(* Logix 5000 AddOnInstructionDefinition export AMP_Point_to_Point_FC; software revision 20.04 *)

TYPE AMP_Status_Word :   // Applied Motion Input Assembly Status Word
STRUCT
   Enabled : BOOL;   // Motor Enabled (Motor Disabled if this bit = 0)
   Sampling : BOOL;   // Sampling (for Quick Tuner)
   Drive_Fault : BOOL;   // Drive Fault (check Alarm Code)
   In_Position : BOOL;   // In Position (motor is in position)
   Moving : BOOL;   // Moving (motor is moving)
   Jogging : BOOL;   // Jogging (currently in jog mode)
   Stopping : BOOL;   // Stopping (in the process of stopping from a stop command)
   Waiting : BOOL;   // Waiting (for an input; executing a WI command)
   Saving : BOOL;   // Saving (parameter data is being saved)
   Alarm_Present : BOOL;   // Alarm present (check Alarm Code)
   Homing : BOOL;   // Homing (executing an SH command)
   Wait_Time : BOOL;   // Waiting (for time; executing a WD or WT command)
   Wizard_Running : BOOL;   // Wizard running (Timing Wizard is running)
   Checking_Encoder : BOOL;   // Checking encoder (Timing Wizard is running)
   Q_Program_Running : BOOL;   // Q Program is running
   Initializing : BOOL;   // Initializing (happens at power up) ; Servo Ready (for SV200 drives only)
END_STRUCT
END_TYPE

TYPE AMP_Input_Assembly_v2 :   // Applied Motion Drive Input Assembly Version 2.0
STRUCT
   Status_Code : DINT;   // Status Code
   Alarm_Code : DINT;   // Alarm Code
   Voltage : DINT;   // Supply Voltage (x0.1V)
   Current : DINT;   // Actual Current (mA)
   Temp : DINT;   // Drive Temperature (0.1 deg C)
   Encoder_Position : DINT;   // Encoder Position (20,000 counts = 1 shaft turn)
   Absolute_Position : DINT;   // Absolute Position (20,000 counts = 1 shaft turn)
   Position_Error : DINT;   // Position Error (counts)
   Actual_Velocity : DINT;   // Actual Velocity (rev/sec * 240, 0 when no encoder)
   Extended_Inputs : DINT;   // Input Status (Extended)
   Main_Board_Inputs : DINT;   // Input Status (Main board)
   Word11 : DINT;   // Reserved
   Analog_Input_1 : DINT;   // Analog Input 1 (ADC counts, 0=min V, 16383 = max V)
   Analog_Input_2 : DINT;   // Analog Input 2 (ADC counts, 0=min V, 16383 = max V)
END_STRUCT
END_TYPE

ADD_ON_INSTRUCTION AMP_Point_to_Point_FC   (* revision 1.0 *)
// Applied Motion - Point to Point Move with Speed Change AOI
// Help:
// The Point-to-Point Move with Speed Change AOI executes a feed to length (relative move) with a speed change after an initial travel distance (FC command).
VAR_IN_OUT
   Input : DINT[14]; {required}   // Drive Input Assembly
   Output : DINT[16]; {required}   // Drive Output Assembly
        [0]   // Command Word
        [1]   // Jog Speed (0.25 rev/min)
        [2]   // Jog Acceleration (10 rev/s/s)
        [3]   // Jog Deceleration (10 rev/s/s)
        [4]   // Point-to-Point Velocity (0.25 rev/min)
        [5]   // Point-to-Point Acceleration (10 rev/s/s)
        [6]   // Point-to-Point Deceleration (10 rev/s/s)
        [7]   // Point-to-Point Distance (Motor steps)
        [9]   // (2x ASCII Letters in 16 lower word)
        [10]   // Data/Register 1
        [11]   // Data/Register 2
END_VAR
VAR_INPUT
   RPI : DINT := 100; {visible}   // Drive Connection Request Packet Interval (milliseconds)
   Start : BOOL; {required}   // Start the Move
   Change_Distance : DINT; {required}   // Change Distance (steps)
   Change_Speed : REAL; {required}   // Velocity Change (rev/s)
   Distance : DINT; {required}   // Distance to Move (steps, negative = reverse)
   Speed : REAL; {required}   // Velocity of Move (rev/min)
   Acc : REAL; {required}   // Acceleration of Move (rev/s/s)
   Dec : REAL; {required}   // Deceleration (rev/s/s)
END_VAR
VAR_OUTPUT
   Sent : BOOL; {access Read Only, visible}   // Move has been sent to drive
   In_Progress : BOOL; {access Read Only, visible}   // Move in progress
   Done : BOOL; {access Read Only, visible}   // Move completed without errors - desired position reached
   Error : BOOL; {access Read Only, visible}   // Move failed to complete - drive not ready or faulted
   State : DINT := 10; {access Read Only}   // Internal state of progress
END_VAR
VAR
   Loc_StatusCode : AMP_Status_Word;
   Loc_CommandOff_Timer : TIMER;   // Timer to make sure command value was 0 before sending a new command
   Loc_CommandOn_Timer : TIMER;   // Timer to make sure command value is set long enough to be sent to drive
   Loc_Input_Assembly : AMP_Input_Assembly_v2; {access None}
   Loc_Start_ONS : BOOL; {access None}
   Loc_ChangeSpeed_Required : BOOL; {access None}
   Loc_ChangeDistance_Required : BOOL; {access None}
END_VAR

ROUTINE Logic   (* ladder *)
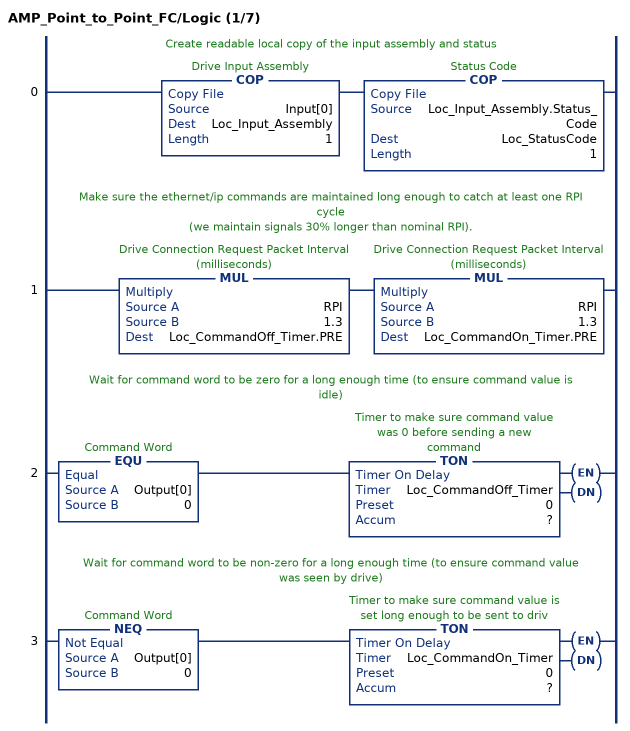
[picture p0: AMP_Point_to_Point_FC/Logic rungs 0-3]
   // Create readable local copy of the input assembly and status
   0: COP(Input[0],Loc_Input_Assembly,1)COP(Loc_Input_Assembly.Status_Code,Loc_StatusCode,1);
   // Make sure the ethernet/ip commands are maintained long enough to catch at least one RPI cycle
   // (we maintain signals 30% longer than nominal RPI).
   1: MUL(RPI,1.3,Loc_CommandOff_Timer.PRE)MUL(RPI,1.3,Loc_CommandOn_Timer.PRE);
   // Wait for command word to be zero for a long enough time (to ensure command value is idle)
   2: EQU(Output[0],0)TON(Loc_CommandOff_Timer,?,?);
   // Wait for command word to be non-zero for a long enough time (to ensure command value was seen by drive)
   3: NEQ(Output[0],0)TON(Loc_CommandOn_Timer,?,?);
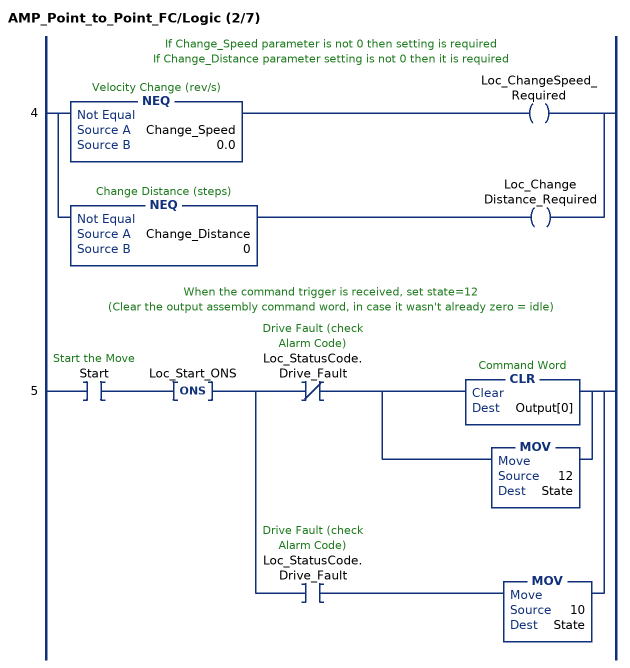
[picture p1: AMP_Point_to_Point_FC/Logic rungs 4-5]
   // If Change_Speed parameter is not 0 then setting is required
   // If Change_Distance parameter setting is not 0 then it is required
   4: [NEQ(Change_Speed,0.0) OTE(Loc_ChangeSpeed_Required) ,NEQ(Change_Distance,0) OTE(Loc_ChangeDistance_Required) ];
   // When the command trigger is received, set state=12
   // (Clear the output assembly command word, in case it wasn't already zero = idle)
   5: XIC(Start)ONS(Loc_Start_ONS)[XIO(Loc_StatusCode.Drive_Fault) [CLR(Output[0]) ,MOV(12,State) ] ,XIC(Loc_StatusCode.Drive_Fault) MOV(10,State) ];
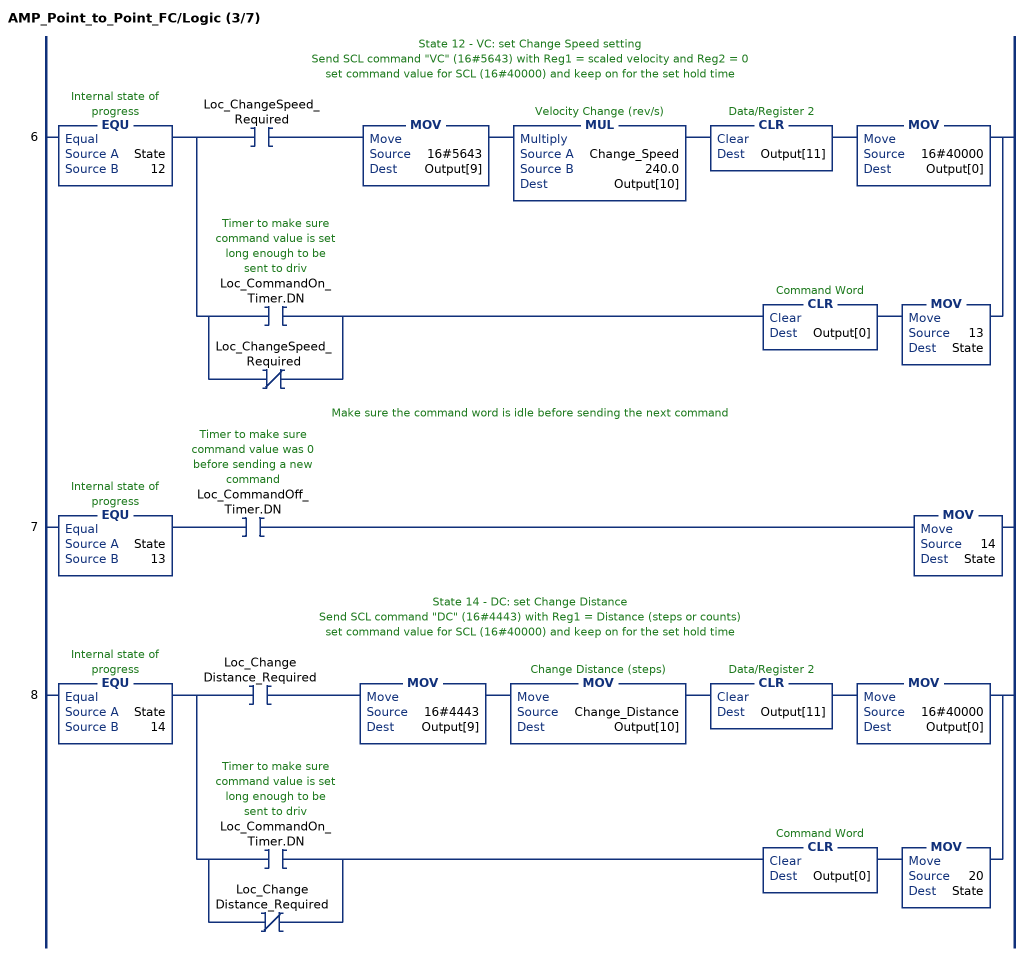
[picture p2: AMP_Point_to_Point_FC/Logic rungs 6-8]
   // State 12 - VC: set Change Speed setting
   // Send SCL command "VC" (16#5643) with Reg1 = scaled velocity and Reg2 = 0
   // set command value for SCL (16#40000) and keep on for the set hold time
   6: EQU(State,12)[XIC(Loc_ChangeSpeed_Required) MOV(16#5643,Output[9]) MUL(Change_Speed,240.0,Output[10]) CLR(Output[11]) MOV(16#40000,Output[0]) ,[XIC(Loc_CommandOn_Timer.DN) ,XIO(Loc_ChangeSpeed_Required) ] CLR(Output[0]) MOV(13,State) ];
   // Make sure the command word is idle before sending the next command
   7: EQU(State,13)XIC(Loc_CommandOff_Timer.DN)MOV(14,State);
   // State 14 - DC: set Change Distance
   // Send SCL command "DC" (16#4443) with Reg1 = Distance (steps or counts)
   // set command value for SCL (16#40000) and keep on for the set hold time
   8: EQU(State,14)[XIC(Loc_ChangeDistance_Required) MOV(16#4443,Output[9]) MOV(Change_Distance,Output[10]) CLR(Output[11]) MOV(16#40000,Output[0]) ,[XIC(Loc_CommandOn_Timer.DN) ,XIO(Loc_ChangeDistance_Required) ] CLR(Output[0]) MOV(20,State) ];
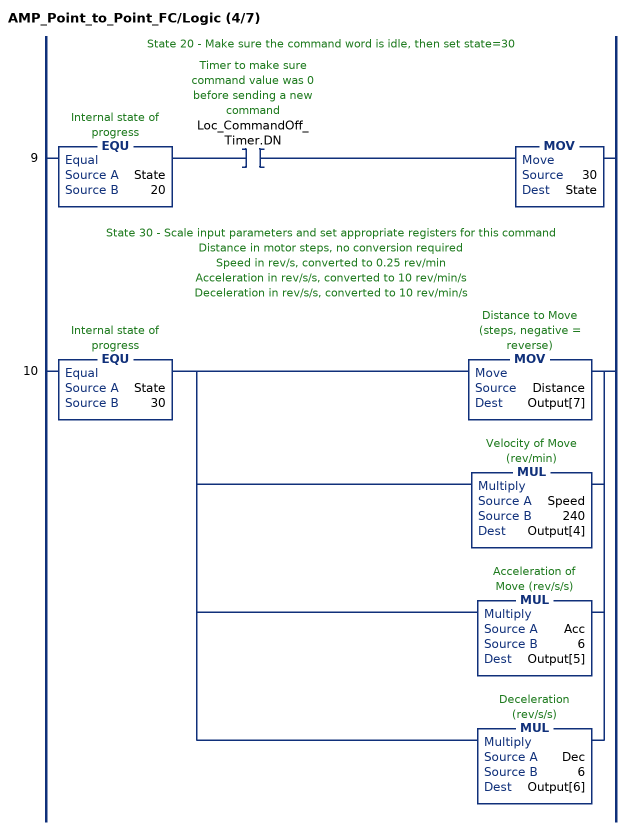
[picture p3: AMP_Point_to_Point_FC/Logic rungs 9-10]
   // State 20 - Make sure the command word is idle, then set state=30
   9: EQU(State,20)XIC(Loc_CommandOff_Timer.DN)MOV(30,State);
   // State 30 - Scale input parameters and set appropriate registers for this command
   // Distance in motor steps, no conversion required
   // Speed in rev/s, converted to 0.25 rev/min
   // Acceleration in rev/s/s, converted to 10 rev/min/s
   // Deceleration in rev/s/s, converted to 10 rev/min/s
   10: EQU(State,30)[MOV(Distance,Output[7]) ,MUL(Speed,240,Output[4]) ,MUL(Acc,6,Output[5]) ,MUL(Dec,6,Output[6]) ];
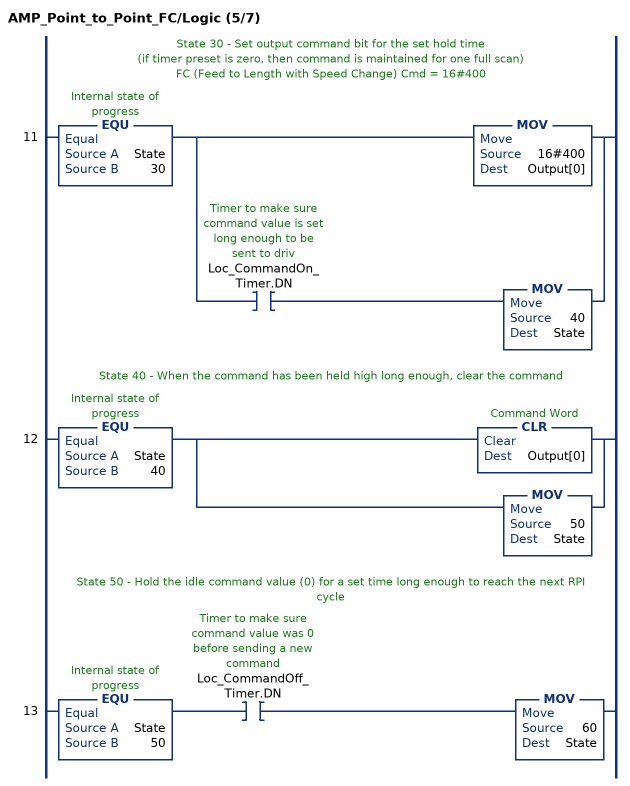
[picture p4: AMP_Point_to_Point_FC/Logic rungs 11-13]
   // State 30 - Set output command bit for the set hold time
   // (if timer preset is zero, then command is maintained for one full scan)
   // FC (Feed to Length with Speed Change) Cmd = 16#400
   11: EQU(State,30)[MOV(16#400,Output[0]) ,XIC(Loc_CommandOn_Timer.DN) MOV(40,State) ];
   // State 40 - When the command has been held high long enough, clear the command
   12: EQU(State,40)[CLR(Output[0]) ,MOV(50,State) ];
   // State 50 - Hold the idle command value (0) for a set time long enough to reach the next RPI cycle
   13: EQU(State,50)XIC(Loc_CommandOff_Timer.DN)MOV(60,State);
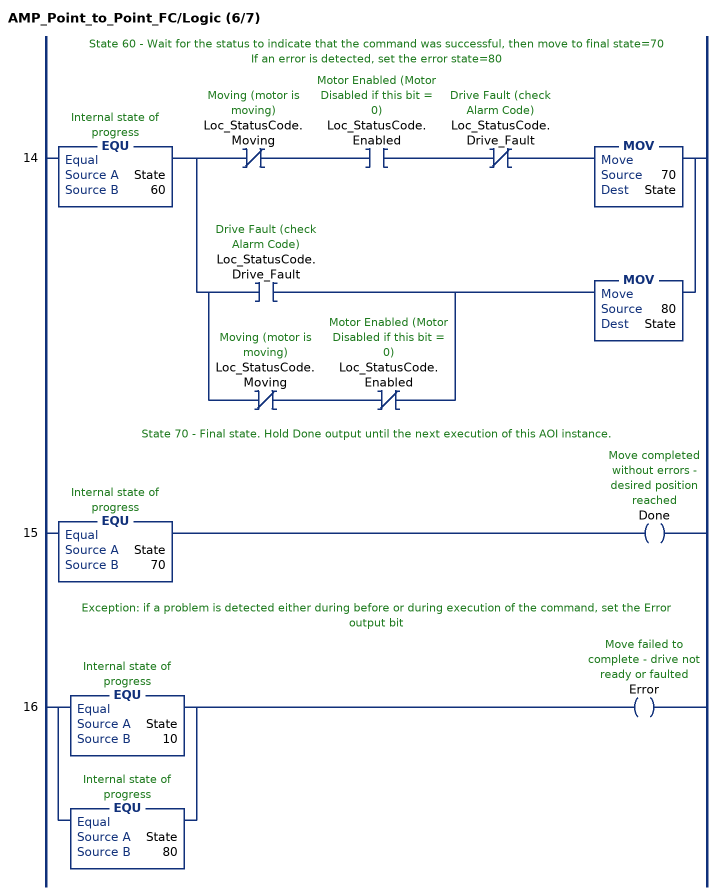
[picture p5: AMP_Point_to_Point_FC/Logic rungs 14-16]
   // State 60 - Wait for the status to indicate that the command was successful, then move to final state=70
   // If an error is detected, set the error state=80
   14: EQU(State,60)[XIO(Loc_StatusCode.Moving) XIC(Loc_StatusCode.Enabled) XIO(Loc_StatusCode.Drive_Fault) MOV(70,State) ,[XIC(Loc_StatusCode.Drive_Fault) ,XIO(Loc_StatusCode.Moving) XIO(Loc_StatusCode.Enabled) ] MOV(80,State) ];
   // State 70 - Final state. Hold Done output until the next execution of this AOI instance.
   15: EQU(State,70)OTE(Done);
   // Exception: if a problem is detected either during before or during execution of the command, set the Error output bit
   16: [EQU(State,10) ,EQU(State,80) ]OTE(Error);
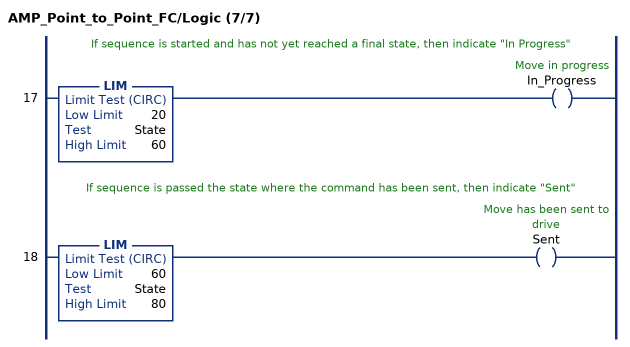
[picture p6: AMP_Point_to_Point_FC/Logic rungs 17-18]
   // If sequence is started and has not yet reached a final state, then indicate "In Progress"
   17: LIM(20,State,60)OTE(In_Progress);
   // If sequence is passed the state where the command has been sent, then indicate "Sent"
   18: LIM(60,State,80)OTE(Sent);
END_ROUTINE
END_ADD_ON_INSTRUCTION
